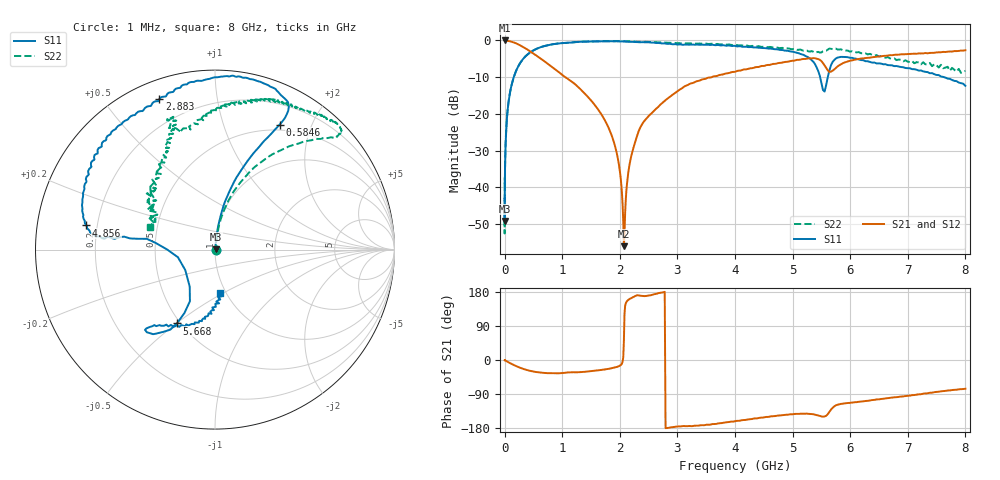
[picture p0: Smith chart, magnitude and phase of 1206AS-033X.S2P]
!s-Parameter Generated by FASTRON Sdn. Bhd.
!FASTRON P/N : 1206AS-033X
!Keysight Technologies: E5071C_MY46733604_B.14.02
!Date: Wed Nov 15 10:01:21 2023
!Version  :Rev00  Wed Nov 15 10:01:21 2023
!Data & Calibration Information:
!Freq  S11:SOLT2(ON)  S21:SOLT2(ON)  S12:SOLT2(ON)  S22:SOLT2(ON)
!PortZ  Port1:50+j0  Port2:50+j0
!When reading reference impedance value at option line is always used.
! Remarks : This data is being provided solely for informational purposes.
# Hz S dB R 50
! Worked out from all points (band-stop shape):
!   1601 points, 1 MHz to 8 GHz, reference 50 ohm
!   highest |S21| = -0.02 dB at 6.301 MHz (marker M1); lowest = -56.0 dB at 2.072 GHz (marker M2)
!   |S21| within 3 dB of the highest: start of sweep to 448 MHz; 7.773 GHz to end of sweep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
!   lowest |S11| = -49.1 dB at 1.505 MHz (marker M3), VSWR 1.01, Z = 50.3 + j0.128 ohm
!   |S11| at or under -10 dB: start of sweep to 160.3 MHz; 5.478 GHz to 5.611 GHz (132.9 MHz wide, 2.4 % of centre); 7.627 GHz to end of sweep
!   |S22| runs from -52.5 to -0.2 dB; largest |S21 - S12| = 0.0069
!   S11 on the Smith chart (normalised r, x): 1 MHz: 1.01, -0.00; 584.6 MHz: 0.43, +1.56; 2.883 GHz: 0.08, +0.69; 4.856 GHz: 0.16, +0.09; 5.668 GHz: 0.48, -0.50; 8 GHz: 0.94, -0.48
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1000000  -46.64 -1.8  -0.03 -0.2  -0.04 -0.2  -48.58 -0.0
1504644  -49.15 21.4  -0.03 -0.2  -0.04 -0.2  -48.33 -0.0
4479405  -39.59 65.4  -0.04 -0.5  -0.04 -0.4  -39.85 69.4
6301378  -36.72 61.6  -0.02 -0.8  -0.03 -0.5  -39.59 70.2
2.00676e7  -27.27 81.5  -0.05 -1.9  -0.07 -1.8  -27.10 80.7
8.994653e7  -14.58 80.7  -0.23 -7.8  -0.24 -7.8  -14.62 78.7
4.006501e8  -3.81 66.2  -2.53 -26.9  -2.54 -27.0  -3.81 57.5
5.846244e8  -2.10 62.6  -4.47 -32.5  -4.49 -32.5  -2.09 50.2
1.249007e9  -0.45 68.7  -12.30 -32.4  -12.30 -32.5  -0.44 42.8
1.7949e9  -0.26 80.7  -23.41 -23.7  -23.43 -23.9  -0.22 45.0
1.92273e9  -0.23 83.8  -29.05 -19.6  -29.09 -20.0  -0.20 45.7
2.007949e9  -0.28 85.8  -36.34 -14.2  -36.50 -14.6  -0.21 46.4
2.071864e9  -0.31 87.5  -56.01 51.5  -56.20 59.2  -0.23 47.3
2.125126e9  -0.34 88.8  -39.07 155.3  -38.95 154.5  -0.28 46.9
2.354847e9  -0.50 95.0  -23.75 169.7  -23.78 169.4  -0.35 49.9
2.883048e9  -0.96 110.2  -15.18 -177.8  -15.23 -178.0  -0.65 56.6
3.95342e9  -1.53 143.5  -8.60 -162.6  -8.61 -162.7  -1.26 72.8
4.856488e9  -2.75 169.4  -5.90 -145.0  -5.87 -145.2  -2.18 89.9
5.33235e9  -5.42 172.6  -4.89 -142.6  -4.86 -143.0  -2.93 99.6
5.668252e9  -6.69 -117.3  -8.51 -130.6  -8.50 -131.1  -2.29 110.4
6.072257e9  -4.93 -130.3  -5.28 -111.6  -5.26 -111.9  -3.11 111.0
8e9  -12.37 -83.4  -2.68 -75.8  -2.66 -76.3  -8.30 160.8
